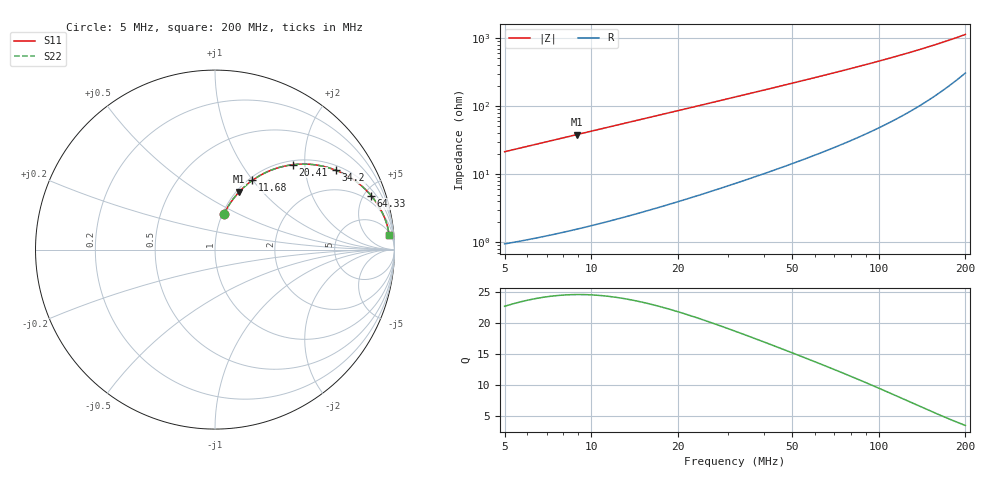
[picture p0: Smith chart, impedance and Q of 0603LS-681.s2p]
# MHz S MA R 50
!Freq  MagS11  AngS11  MagS21  AngS21  MagS12  AngS12  MagS22  AngS22
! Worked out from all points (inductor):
!   801 points, 5 MHz to 200 MHz, reference 50 ohm
!   read as one part in series: L = 677 nH near 5.093 MHz
!   highest Q = 24.5 at 8.898 MHz (marker M1), where L = 677 nH
!   S11 on the Smith chart (normalised r, x): 5 MHz: 1.02, +0.43; 11.68 MHz: 1.04, +0.99; 20.41 MHz: 1.08, +1.74; 34.2 MHz: 1.16, +2.93; 64.33 MHz: 1.43, +5.61; 200 MHz: 7, +22
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5  0.2063 75.6  0.9694 -11.9  0.9694 -11.9  0.2063 75.6
6.809928  0.2753 71.7  0.95 -16.0  0.95 -16.0  0.2753 71.7
8.897989  0.3495 67.2  0.9228 -20.4  0.9228 -20.4  0.3495 67.2
11.68003  0.4381 61.7  0.881 -26.0  0.881 -26.0  0.4381 61.7
13.53712  0.4905 58.2  0.851 -29.3  0.851 -29.3  0.4905 58.2
15.6173  0.5431 54.7  0.8165 -32.9  0.8165 -32.9  0.5431 54.7
20.40588  0.6419 47.5  0.7377 -39.9  0.7377 -39.9  0.6419 47.5
23.75967  0.6954 43.2  0.6858 -44.0  0.6858 -44.0  0.6954 43.2
27.03413  0.7379 39.6  0.6387 -47.5  0.6387 -47.5  0.7379 39.6
30.4775  0.7741 36.4  0.5936 -50.6  0.5936 -50.6  0.7741 36.4
34.20139  0.8056 33.3  0.5496 -53.6  0.5496 -53.6  0.8056 33.3
37.50553  0.8284 30.9  0.5145 -55.8  0.5145 -55.8  0.8284 30.9
43.06977  0.8586 27.5  0.4629 -59.0  0.4629 -59.0  0.8586 27.5
49.23197  0.8832 24.5  0.4149 -61.8  0.4149 -61.8  0.8832 24.5
56.27583  0.9037 21.6  0.3695 -64.4  0.3695 -64.4  0.9037 21.6
64.32748  0.9206 19.0  0.327 -66.6  0.327 -66.6  0.9206 19.0
70.21752  0.9299 17.5  0.3009 -68.0  0.3009 -68.0  0.9299 17.5
84.83031  0.946 14.4  0.2493 -70.4  0.2493 -70.4  0.946 14.4
102.9578  0.9577 11.6  0.2029 -72.2  0.2029 -72.2  0.9577 11.6
135.1485  0.9679 8.4  0.1479 -73.3  0.1479 -73.3  0.9679 8.4
167.8542  0.972 6.3  0.1115 -72.3  0.1115 -72.3  0.972 6.3
200  0.9731 4.8  0.08644 -69.5  0.08644 -69.5  0.9731 4.8
